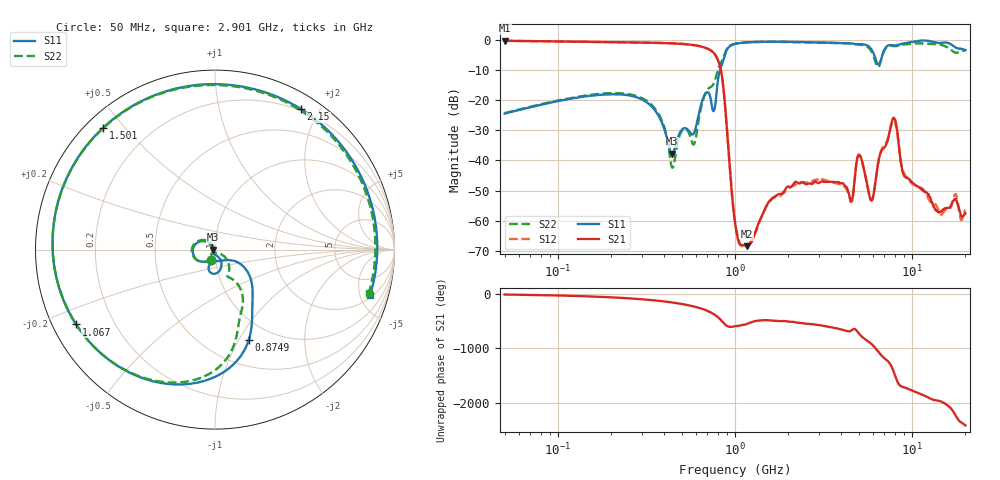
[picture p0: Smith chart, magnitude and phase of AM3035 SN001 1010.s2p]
# Hz S DB R 50
!freq MagS11 AngS11 MagS21 AngS21 MagS12 AngS12 MagS22 AngS22
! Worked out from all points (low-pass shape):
!   1601 points, 50 MHz to 20.05 GHz, reference 50 ohm
!   highest |S21| = -0.37 dB at 50 MHz (marker M1); lowest = -68.4 dB at 1.167 GHz (marker M2)
!   |S21| within 3 dB of the highest: start of sweep to 721.9 MHz
!   lowest |S11| = -37.8 dB at 440.8 MHz (marker M3), VSWR 1.03, Z = 48.7 - j0.0395 ohm
!   |S11| at or under -10 dB: start of sweep to 824 MHz
!   |S22| runs from -42.4 to -0.7 dB; largest |S21 - S12| = 0.0068
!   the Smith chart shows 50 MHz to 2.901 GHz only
!   S11 on the Smith chart (normalised r, x): 50 MHz: 0.95, -0.11; 874.9 MHz: 0.78, -1.10; 1.067 GHz: 0.07, -0.25; 1.501 GHz: 0.05, +0.44; 2.15 GHz: 0.18, +1.77; 2.901 GHz: 2.32, -6.17
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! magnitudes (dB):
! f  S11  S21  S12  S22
! 50 MHz  -24.5  -0.4  -0.4  -24.3
! 135.9 MHz  -19.0  -0.7  -0.7  -18.7
! 369.6 MHz  -25.1  -1.1  -1.1  -24.5
! 440.8 MHz  -37.8  -1.2  -1.2  -42.2
! 685.8 MHz  -17.7  -2.8  -2.8  -17.4
! 756 MHz  -23.7  -4.3  -4.3  -14.8
! 874.9 MHz  -5.4  -20.2  -20.1  -4.7
! 1.005 GHz  -1.4  -61.3  -60.9  -1.3
! 1.067 GHz  -1.1  -67.8  -67.7  -1.1
! 1.167 GHz  -0.9  -68.4  -67.9  -0.9
! 1.501 GHz  -0.7  -55.3  -55.3  -0.7
! 2.15 GHz  -0.7  -47.7  -48.3  -0.8
! 2.722 GHz  -0.9  -47.8  -47.0  -1.0
! 2.901 GHz  -0.9  -47.3  -46.3  -1.0
! 4.531 GHz  -1.3  -53.5  -53.8  -1.3
! 5.051 GHz  -1.5  -38.3  -38.1  -1.7
! 5.912 GHz  -3.2  -53.3  -53.3  -3.9
! 7.402 GHz  -1.8  -31.8  -31.9  -2.1
! 7.978 GHz  -2.0  -26.2  -27.1  -2.2
! 9.061 GHz  -1.2  -45.3  -44.6  -1.6
! 14.42 GHz  -1.1  -57.1  -57.7  -1.6
! 20.05 GHz  -3.4  -57.6  -56.4  -3.6
